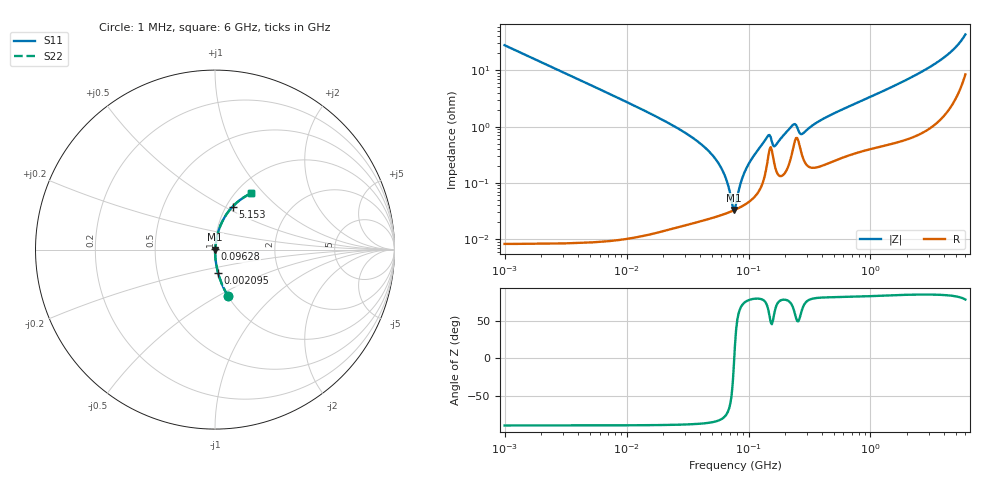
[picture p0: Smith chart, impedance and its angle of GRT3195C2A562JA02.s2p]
!Murata Part Number: GRT3195C2A562JA02
!These Parameters are Measured in Series Mode Connection
!Data Generated on Jun 19, 2026
!  o--ll--o
!Port1  Port2
!  o------o
!Operation Temp=25[degC], DC Bias Voltage=0[V]
!Freq. Start=1000[kHz] Stop=6[GHz] 401[Steps]
# Hz S RI R 50
!Freq.(Hz) S11(Real) S11(Imag) S21(Real) S21(Imag) S12(Real) S12(Imag) S22(Real) S22(Imag)
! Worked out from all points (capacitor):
!   401 points, 1 MHz to 6 GHz, reference 50 ohm
!   read as one part in series: C = 5.7 nF near 1.044 MHz
!   lowest |Z| = 33 mohm at 75.79 MHz (marker M1)
!   series resonance near 76.34 MHz, so ESL is about 760 pH
!   S11 on the Smith chart (normalised r, x): 1 MHz: 1.00, -0.56; 2.095 MHz: 1.00, -0.27; 96.28 MHz: 1.00, +0.00; 5.153 GHz: 1.07, +0.55; 6 GHz: 1.17, +0.85
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1000000  0.0724 -0.2591  0.9276 0.2591  0.9276 0.2591  0.0724 -0.2591
2094801  0.0175 -0.1309  0.9825 0.1309  0.9825 0.1309  0.0175 -0.1309
4293785  0.00427 -0.0646  0.9957 0.0646  0.9957 0.0646  0.00427 -0.0646
1.843659e7  0.000335 -0.0142  0.9997 0.0142  0.9997 0.0142  0.000335 -0.0142
3.389622e7  0.000231 -0.0066  0.9998 0.0066  0.9998 0.0066  0.000231 -0.0066
5.013812e7  0.000247 -0.00317  0.9998 0.00317  0.9998 0.00317  0.000247 -0.00317
6.23192e7  0.000278 -0.00151  0.9997 0.00151  0.9997 0.00151  0.000278 -0.00151
7.57932e7  0.000326 -5.32e-05  0.9997 5.32e-05  0.9997 5.32e-05  0.000326 -5.32e-05
7.745967e7  0.000333 0.000109  0.9997 -0.000109  0.9997 -0.000109  0.000333 0.000109
8.825674e7  0.000384 0.0011  0.9996 -0.0011  0.9996 -0.0011  0.000384 0.0011
9.627852e7  0.000432 0.00179  0.9996 -0.00179  0.9996 -0.00179  0.000432 0.00179
1.424119e8  0.00229 0.0062  0.9977 -0.0062  0.9977 -0.0062  0.00229 0.0062
1.487431e8  0.00395 0.00587  0.996 -0.00587  0.996 -0.00587  0.00395 0.00587
1.658303e8  0.00186 0.00418  0.9981 -0.00418  0.9981 -0.00418  0.00186 0.00418
2.297971e8  0.00381 0.00985  0.9962 -0.00985  0.9962 -0.00985  0.00381 0.00985
2.400133e8  0.00564 0.0095  0.9944 -0.0095  0.9944 -0.0095  0.00564 0.0095
2.734687e8  0.00324 0.00658  0.9968 -0.00658  0.9968 -0.00658  0.00324 0.00658
3.325952e8  0.00196 0.0102  0.998 -0.0102  0.998 -0.0102  0.00196 0.0102
1.428092e9  0.00707 0.0475  0.9929 -0.0475  0.9929 -0.0475  0.00707 0.0475
3.193267e9  0.0237 0.1166  0.9763 -0.1166  0.9763 -0.1166  0.0237 0.1166
5.152685e9  0.0981 0.2394  0.9019 -0.2394  0.9019 -0.2394  0.0981 0.2394
6e9  0.2012 0.3134  0.7988 -0.3134  0.7988 -0.3134  0.2012 0.3134
